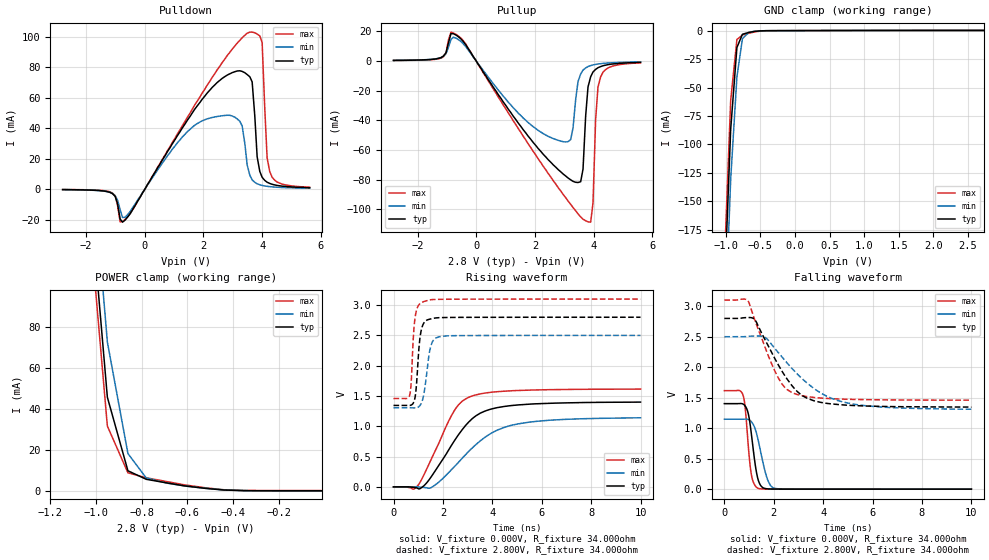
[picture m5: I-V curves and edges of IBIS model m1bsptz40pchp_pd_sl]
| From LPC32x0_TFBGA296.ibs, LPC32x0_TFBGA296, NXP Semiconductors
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| |   Rev 0.20 IBIS Model Design Automation Generation   |
| |   N O N - S I L I C O N   C O R R E L A T E D   |
| |   This IBIS [Model] is pre-Beta tactical support   |
| |  Note: this IBIS [Model] contains clamp curves generated   |
| |   through simulation which should not be relied upon   |
| mem1bsptz40pchp
|   Bidirectional Pad 2.8
|   3state Output
|   Plain Input
|   1ns Slew Rate control
|   CMOS
| Pull Down Mode (p1=1, p2=1)
[Model]   m1bsptz40pchp_pd_sl | of mem1bsptz40pchp
Model_type   I/O
Polarity   Non-Inverting
Enable   Active-Low
|  Reciever Thresholds
Vinl   = 0.36V
Vinh   = 0.84V
| AC Test Load Conditions
Vref   = 0
Cref   = 1.2e-11
Rref   = 1000000000
Vmeas   = 0.6
| [Process Range]   typical   min   max
| C_comp edge width   400.000ps   400.000ps   400.000ps
| C_comp Tstrobe   40.000fs   40.000fs   40.000fs
C_comp   2.018pF   1.942pF   2.107pF
[Temperature Range]   25   125   -40
[Voltage Range]   2.80V   2.50V   3.10V
[GND Clamp Reference]   0.00V   0.00V   0.00V
[Pulldown Reference]   0.00V   0.00V   0.00V
[POWER Clamp Reference]   2.80V   2.50V   3.10V
[Pullup Reference]   2.80V   2.50V   3.10V
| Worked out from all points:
|   slope of the pulldown table from 0 to 0.42 V, typ, clamps not added: 31 ohm
|   slope of the pullup table from 0 to 0.42 V, typ, clamps not added: 32.8 ohm
|   GND clamp passes 1 mA (typ) near -0.61 V on its own axis
|   POWER clamp passes 1 mA (typ) near -0.49 V on its own axis
|   rising waveform, V_fixture 0.000V, R_fixture 34.000ohm: 20-80 % time 1.46ns typ, 1.87ns min, 1.14ns max; typ from 0 V to 1.4 V
|   falling waveform, V_fixture 0.000V, R_fixture 34.000ohm: 20-80 % time 277ps typ, 392ps min, 209ps max; typ from 1.4 V to 0 V
|   rising waveform, V_fixture 2.800V, R_fixture 34.000ohm: 20-80 % time 170ps typ, 240ps min, 142ps max; typ from 1.34 V to 2.8 V
|   falling waveform, V_fixture 2.800V, R_fixture 34.000ohm: 20-80 % time 1.29ns typ, 1.89ns min, 1ns max; typ from 2.8 V to 1.35 V
[GND Clamp]
| ref voltage   0.00V   0.00V   0.00V
|   Voltage   I(typ)   I(min)   I(max)
-2.8V     -3.643A    -3.653A    -3.644A
-1.01V    -211.8mA   -255.9mA   -186.6mA
-930mV    -86.6mA    -130.6mA   -61.24mA
-840mV    -14.83mA   -40.64mA   -7.829mA
-760mV    -3.203mA   -7.088mA   -3.83mA
-670mV    -1.622mA   -1.69mA    -2.382mA
-500mV    -233.9uA   -204.7uA   -414uA
2.73V     154.6uA    78.63uA    263.6uA
[Power Clamp]   | Vtable = Vcc - Vpad
| ref voltage   2.80V   2.50V   3.10V
|   Voltage   I(typ)   I(min)   I(max)
-2.82V    3.531A     3.518A     3.546A
-1.03V    149.7mA    178.4mA    134.4mA
-950mV    45.73mA    72.62mA    31.68mA
-860mV    9.888mA    18.31mA    8.901mA
-780mV    5.742mA    6.415mA    6.476mA
-690mV    3.983mA    3.877mA    4.635mA
-610mV    2.503mA    2.443mA    2.981mA
-440mV    510.7uA    586.4uA    642.9uA
-270mV    156.9uA    89.28uA    264.9uA
-10mV     154.6uA    73.24uA    264uA
[Pulldown]
| ref voltage   0.00V   0.00V   0.00V
|   Voltage   I(typ)   I(min)   I(max)
-2.8V     -319.3uA   -345.4uA   -253.1uA
-1.18V    -2.159mA   -2.186mA   -1.786mA
-670mV    -20.28mA   -18.52mA   -19.91mA
1.11V     35.01mA    30.34mA    36.12mA
2.13V     63.07mA    46.11mA    68.26mA
3.24V     77.61mA    44.53mA    97.58mA
3.66V     70.35mA    6.093mA    103mA
3.83V     21.24mA    3.51mA     101.7mA
4V        7.762mA    2.426mA    96.16mA
4.17V     4.525mA    1.839mA    20.54mA
4.26V     3.73mA     1.638mA    11.44mA
5.62V     952.8uA    583.3uA    1.27mA
[Pullup]   | Vtable = Vcc - Vpad
| ref voltage   2.80V   2.50V   3.10V
|   Voltage   I(typ)   I(min)   I(max)
-2.82V    285.7uA    306.1uA    228.4uA
-520mV    14.73mA    12.99mA    15.29mA
2.79V     -73.12mA   -53.48mA   -85.2mA
3.22V     -80.05mA   -52.98mA   -96.52mA
3.47V     -81.85mA   -13.92mA   -103mA
3.64V     -72.85mA   -6.25mA    -106.5mA
3.81V     -17.56mA   -3.872mA   -108.3mA
3.9V      -10.74mA   -3.234mA   -108.5mA
3.98V     -7.509mA   -2.77mA    -95.67mA
4.07V     -5.754mA   -2.418mA   -39.4mA
4.24V     -3.885mA   -1.924mA   -10.82mA
5.6V      -1.045mA   -712.7uA   -1.372mA
[Ramp]
R_load   = 34.000ohm
|   dV/dt(typ)   dV/dt(min)   dV/dt(max)
dV/dt_r   969.889mV/1.305ns   805.310mV/1.665ns   1.109V/1.035ns
dV/dt_f   1.001V/1.120ns   838.492mV/1.635ns   1.123V/875.000ps
[Rising Waveform]  | cubic spline decimation from 2001 points
V_fixture   = 0.000V
R_fixture   = 34.000ohm
|   Time   V(typ)   V(min)   V(max)
0s        4.292nV    139.7nV    2.459nV
810ps     -7.213mV   186uV      -37.6mV
975ps     -22.56mV   -1.932mV   16.58mV
1.53ns    168.7mV    -10.11mV   458.1mV
2.46ns    757.9mV    331.6mV    1.257V
2.765ns   935.1mV    465.3mV    1.408V
3.175ns   1.121V     637.3mV    1.499V
4.145ns   1.303V     925.6mV    1.569V
5.065ns   1.353V     1.041V     1.591V
10ns      1.399V     1.14V      1.614V
[Falling Waveform]  | cubic spline decimation from 2001 points
V_fixture   = 0.000V
R_fixture   = 34.000ohm
|   Time   V(typ)   V(min)   V(max)
0s        1.402V     1.147V     1.615V
750ps     1.397V     1.147V     1.548V
845ps     1.362V     1.148V     1.327V
965ps     1.241V     1.141V     727.8mV
1.08ns    947.2mV    1.111V     270.3mV
1.25ns    400.1mV    983.7mV    55.5mV
1.365ns   158.7mV    810mV      14.51mV
1.74ns    5.787mV    167.6mV    1.787mV
2.035ns   1.79mV     14.44mV    1.113mV
10ns      7.524uV    12.08uV    6.851uV
[Rising Waveform]  | cubic spline decimation from 2001 points
V_fixture   = 2.800V
V_fixture_min = 2.500V
V_fixture_max = 3.100V
R_fixture   = 34.000ohm
|   Time   V(typ)   V(min)   V(max)
0s        1.344V     1.305V     1.458V
660ps     1.344V     1.305V     1.522V
720ps     1.351V     1.304V     1.753V
825ps     1.402V     1.303V     2.6V
910ps     1.594V     1.304V     2.878V
1.065ns   2.438V     1.339V     3.022V
1.19ns    2.674V     1.457V     3.052V
1.51ns    2.772V     2.323V     3.088V
1.845ns   2.792V     2.475V     3.094V
10ns      2.799V     2.499V     3.099V
[Falling Waveform]  | cubic spline decimation from 2001 points
V_fixture   = 2.800V
V_fixture_min = 2.500V
V_fixture_max = 3.100V
R_fixture   = 34.000ohm
|   Time   V(typ)   V(min)   V(max)
0s        2.799V     2.499V     3.099V
965ps     2.813V     2.505V     3.081V
1.255ns   2.767V     2.511V     2.748V
1.65ns    2.446V     2.487V     2.323V
2.065ns   2.124V     2.296V     1.919V
2.36ns    1.916V     2.154V     1.71V
2.75ns    1.69V      1.973V     1.581V
3.615ns   1.45V      1.654V     1.504V
4.845ns   1.38V      1.425V     1.475V
10ns      1.346V     1.31V      1.459V
